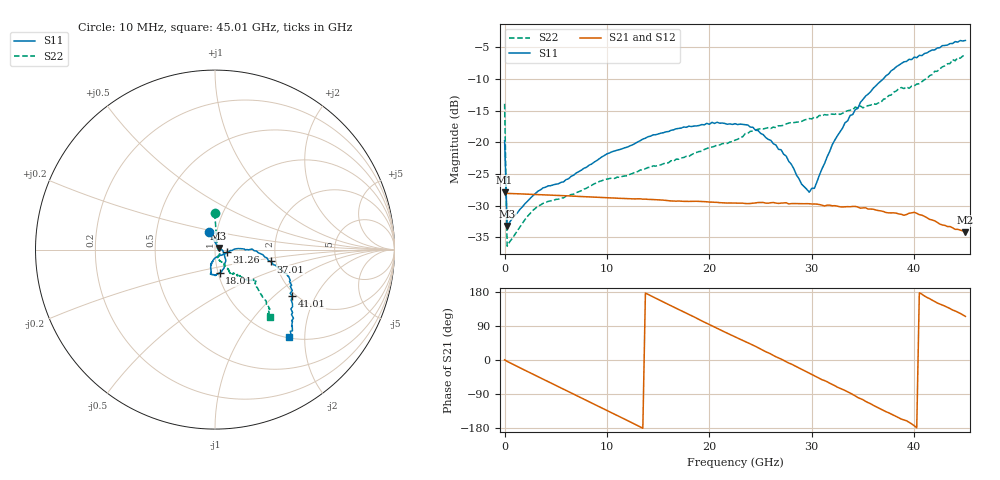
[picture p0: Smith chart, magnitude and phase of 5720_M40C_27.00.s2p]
! Device:  ADRF5720
! Description: 0.5dB LSB GaAs MMIC 6-bit Digital Attenuator
! Frequency:  0.000009 -  40 GHz
! Ports:
!	RF1	= Port 1
!	RF2	= Port 2
! Vdd:  3.3 Volt
! Vss:  -3.3 Volt
! Control:  0/3.3 Volt
! State:  27.00 dB attenuation
! Data:  The device was measured using G-S-G Probes on a matrix board.
!  Data was collected using an calibrated 4 port network analyzer.
!  The reference plane for this measurement is at the launchers.
! Note:  Analog Devices supplies this data as a sample of measured data
!  for this product.  Your particular data for this product may vary.
!  Data was taken at -40 degrees C.
!  Analog Devices reserves the right to change this data at anytime.
# GHZ S DB R 45.0
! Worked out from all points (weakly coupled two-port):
!   181 points, 10 MHz to 45.01 GHz, reference 45 ohm
!   highest |S21| = -27.88 dB at 10 MHz (marker M1); lowest = -34.2 dB at 45.01 GHz (marker M2)
!   lowest |S11| = -33.2 dB at 260 MHz (marker M3), VSWR 1.04, Z = 46.8 + j0.914 ohm
!   |S11| at or under -10 dB: start of sweep to 36.97 GHz
!   |S22| runs from -36.4 to -6.3 dB; largest |S21 - S12| = 0.00018
!   S11 on the Smith chart (normalised r, x): 10 MHz: 0.92, +0.18; 18.01 GHz: 1.02, -0.27; 31.26 GHz: 1.14, -0.03; 37.01 GHz: 1.88, -0.28; 41.01 GHz: 1.91, -1.33; 45.01 GHz: 1.02, -1.67
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0.01  -19.74 109.5  -27.88 0.4  -27.90 0.5  -13.90 90.4
0.26  -33.18 26.4  -28.05 -3.7  -28.07 -3.7  -36.38 33.1
3.26  -27.70 -4.6  -28.24 -43.9  -28.26 -44.0  -30.04 -32.1
5.76  -26.23 -18.4  -28.41 -77.0  -28.43 -77.0  -28.75 -52.0
7.76  -24.08 -32.3  -28.56 -103.5  -28.58 -103.5  -27.38 -65.8
10.01  -21.80 -43.1  -28.73 -133.3  -28.75 -133.3  -25.79 -69.9
15.26  -18.54 -67.0  -29.07 156.2  -29.09 156.2  -23.54 -67.3
18.01  -17.43 -79.0  -29.31 120.3  -29.33 120.3  -22.23 -62.1
22.76  -17.18 -99.1  -29.59 57.9  -29.61 57.9  -19.51 -58.9
24.26  -17.61 -100.3  -29.60 39.3  -29.62 39.2  -18.22 -57.3
26.01  -19.68 -103.7  -29.52 15.8  -29.54 15.7  -17.79 -56.5
27.51  -22.16 -101.9  -29.52 -4.9  -29.55 -5.0  -17.08 -57.1
29.01  -26.58 -90.5  -29.68 -24.2  -29.70 -24.4  -16.68 -57.4
29.76  -27.86 -63.8  -29.68 -34.5  -29.71 -34.7  -16.23 -57.7
30.26  -27.25 -43.0  -29.72 -41.2  -29.75 -41.4  -15.98 -56.9
31.26  -23.31 -11.9  -30.03 -54.4  -30.06 -54.5  -15.60 -54.8
33.26  -16.88 2.1  -30.17 -80.5  -30.18 -80.6  -15.14 -51.7
37.01  -9.94 -12.0  -30.91 -133.4  -30.93 -133.6  -13.18 -45.1
37.76  -8.69 -16.2  -31.13 -142.4  -31.16 -142.5  -12.51 -44.7
41.01  -5.96 -31.1  -31.67 169.0  -31.68 168.8  -10.09 -42.2
43.76  -4.38 -44.6  -33.48 131.9  -33.52 131.6  -6.91 -47.4
45.01  -3.90 -49.8  -34.17 115.1  -34.23 115.0  -6.31 -50.7
